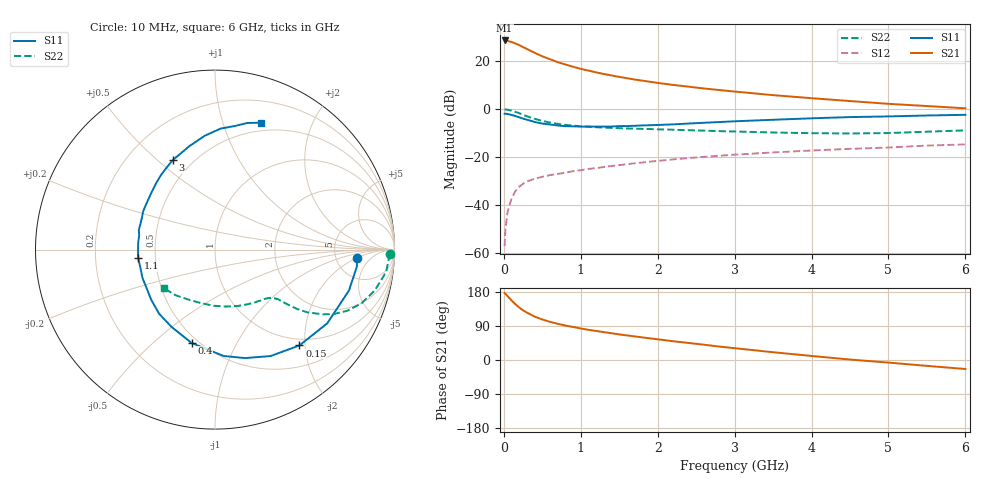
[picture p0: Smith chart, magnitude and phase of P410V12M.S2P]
! SIEMENS Small Signal Semiconductors
! BFP182
! Si NPN RF Bipolar Junction Transistor in SOT143
! VCE = 10 V  IC = 12 mA
! Common Emitter S-Parameters:  March  1996
# GHz  S  MA  R  50
!  f  S11  S21  S12  S22
! GHz  MAG  ANG  MAG  ANG  MAG  ANG  MAG  ANG
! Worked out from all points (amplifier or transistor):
!   36 points, 10 MHz to 6 GHz, reference 50 ohm
!   highest |S21| = 28.4 dB at 10 MHz (marker M1)
!   |S21| within 3 dB of that: start of sweep to 265.6 MHz
!   unconditionally stable (mu >= 1): 1.202 GHz to 5.744 GHz
!   at 250 MHz: K = 0.34, MSG = 28.4 dB, |S12| = -31.1 dB
!   at 1.4 GHz: K = 1.05, MAG = 17.4 dB, |S12| = -23.8 dB
!   at 6 GHz: K = 0.98, MSG = 7.5 dB, |S12| = -14.8 dB
!   S11 on the Smith chart (normalised r, x): 10 MHz: 8.15, -1.94; 150 MHz: 0.87, -1.89; 400 MHz: 0.46, -0.67; 1.1 GHz: 0.40, -0.05; 3 GHz: 0.39, +0.56; 6 GHz: 0.41, +1.35
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0.01  0.7921 -3.2  26.45 176.7  0.0014 74.4  0.9743 -1.4
0.02  0.7962 -6.8  26.43 175.0  0.0031 83.4  0.9701 -2.9
0.05  0.7807 -16.9  25.87 168.1  0.0074 82.8  0.9617 -7.4
0.1  0.7482 -33.3  24.55 157.3  0.0136 71.9  0.9194 -14.3
0.15  0.7117 -48.6  22.87 147.3  0.0195 66.2  0.8689 -20.2
0.2  0.6692 -62.4  21.19 138.5  0.024 62.0  0.8123 -24.8
0.25  0.6272 -74.5  19.25 131.0  0.0278 57.3  0.7544 -28.4
0.3  0.5946 -85.4  17.6 125.1  0.0309 54.1  0.7025 -30.9
0.4  0.5364 -104.0  14.66 114.7  0.0353 49.7  0.6224 -34.2
0.5  0.4942 -119.3  12.37 106.9  0.0387 47.5  0.5627 -35.9
0.6  0.4738 -131.2  10.78 100.7  0.042 46.2  0.5187 -36.8
0.7  0.4522 -141.8  9.348 95.5  0.0445 46.1  0.4885 -37.4
0.9  0.4336 -158.9  7.521 87.1  0.0507 45.8  0.4491 -38.2
1.1  0.4306 -173.6  6.252 79.6  0.0564 45.8  0.425 -39.6
1.3  0.4297 175.0  5.305 73.5  0.0619 45.8  0.4083 -41.2
1.6  0.4395 160.7  4.34 64.9  0.0708 45.4  0.3917 -44.4
2.2  0.4764 138.0  3.152 49.5  0.089 42.8  0.369 -53.0
3  0.5519 115.1  2.293 31.2  0.1117 37.2  0.3389 -68.0
3.5  0.5938 103.9  1.93 20.5  0.1243 32.9  0.323 -79.1
4.5  0.6751 87.3  1.455 1.2  0.1476 25.1  0.3081 -104.7
5.5  0.7286 75.6  1.146 -15.5  0.1726 18.1  0.3356 -130.6
6  0.7525 69.9  1.028 -23.8  0.1827 13.5  0.3575 -143.1
